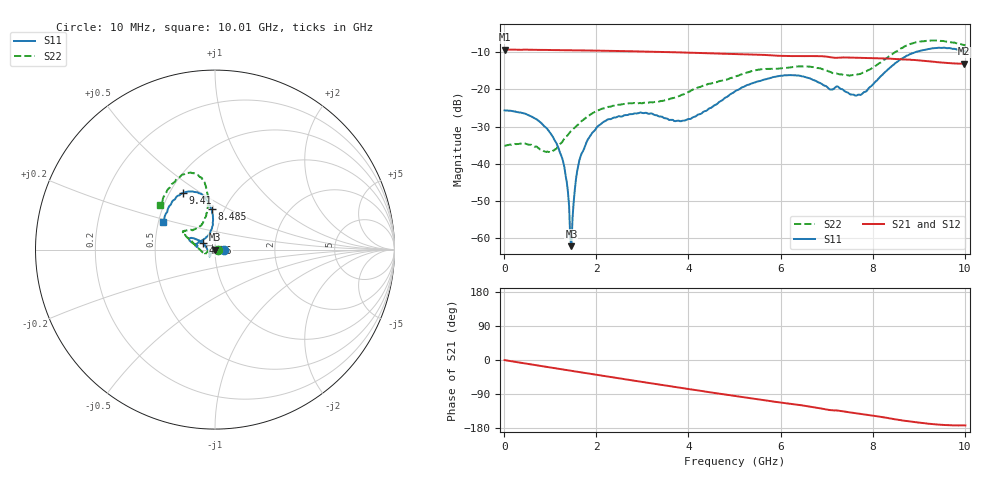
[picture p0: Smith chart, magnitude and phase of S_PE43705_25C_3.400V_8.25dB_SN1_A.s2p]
! Device ID: PE43705
! Serial: 1
! Insertion: A
! Impedance: 50 ohm
! Temp: 25C
! VDD: 3.400V
! Attenuation Step: 8.25dB
#  Hz  S  RI  R  50
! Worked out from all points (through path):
!   401 points, 10 MHz to 10.01 GHz, reference 50 ohm
!   highest |S21| = -9.26 dB at 10 MHz (marker M1); lowest = -13.1 dB at 9.985 GHz (marker M2)
!   group delay of S21, straight-line fit = 49.8 ps
!   lowest |S11| = -62.1 dB at 1.46 GHz (marker M3), VSWR 1.00, Z = 49.9 - j0.0264 ohm
!   |S11| at or under -10 dB: start of sweep to 8.915 GHz
!   |S22| runs from -36.9 to -6.8 dB; largest |S21 - S12| = 0.003
!   S11 on the Smith chart (normalised r, x): 10 MHz: 1.11, -0.00; 4.76 GHz: 0.88, +0.06; 8.485 GHz: 0.87, +0.41; 9.41 GHz: 0.58, +0.42; 10.01 GHz: 0.53, +0.18
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1e7  0.0523 -2.85e-05  0.3443 -0.00154  0.3446 -0.00159  0.0176 0.00025
6.6e8  0.0381 0.0154  0.3321 -0.0772  0.332 -0.0769  0.0073 0.0153
1.085e9  0.018 0.0114  0.3149 -0.1231  0.3149 -0.1231  -0.0108 0.0108
1.31e9  0.00691 0.00548  0.304 -0.1461  0.3041 -0.1459  -0.0211 0.00562
1.41e9  0.00182 0.00198  0.2983 -0.1561  0.2985 -0.1559  -0.0255 0.00278
1.46e9  -0.000737 -0.000265  0.2953 -0.1608  0.2955 -0.1608  -0.0279 0.000586
1.485e9  -0.00153 -0.00113  0.2939 -0.1633  0.294 -0.1632  -0.0286 -0.000221
1.585e9  -0.00675 -0.00439  0.2874 -0.1727  0.2876 -0.1726  -0.0327 -0.00344
1.685e9  -0.0107 -0.00901  0.2811 -0.1818  0.2811 -0.1817  -0.0372 -0.00696
2.21e9  -0.0251 -0.0288  0.2423 -0.2255  0.2424 -0.2253  -0.0525 -0.0223
3.36e9  -0.0292 -0.0323  0.1368 -0.2889  0.1371 -0.2886  -0.0665 -0.0167
3.885e9  -0.0368 -0.00997  0.0841 -0.3022  0.0845 -0.302  -0.0853 0.000805
4.76e9  -0.0651 0.035  -0.00223 -0.3021  -0.00151 -0.3022  -0.1265 0.043
5.01e9  -0.0817 0.0475  -0.0256 -0.2979  -0.0251 -0.2982  -0.1394 0.0537
5.985e9  -0.1378 0.0648  -0.1061 -0.263  -0.1045 -0.2632  -0.1679 0.0915
6.685e9  -0.1303 0.0398  -0.1566 -0.2329  -0.1565 -0.2327  -0.1707 0.1043
7.685e9  -0.0483 0.0703  -0.2081 -0.1673  -0.2079 -0.1673  -0.0734 0.1424
8.36e9  -0.012 0.1935  -0.2332 -0.1148  -0.232 -0.1158  -0.0398 0.2784
8.485e9  -0.0192 0.2241  -0.2358 -0.1028  -0.2344 -0.1043  -0.0434 0.3148
9.41e9  -0.179 0.3158  -0.2296 -0.0386  -0.2288 -0.0386  -0.185 0.4164
9.985e9  -0.2831 0.1631  -0.22 -0.0284  -0.2208 -0.0294  -0.2966 0.2586
1.001e10  -0.2894 0.1543  -0.2212 -0.0286  -0.2217 -0.0299  -0.3039 0.2478
